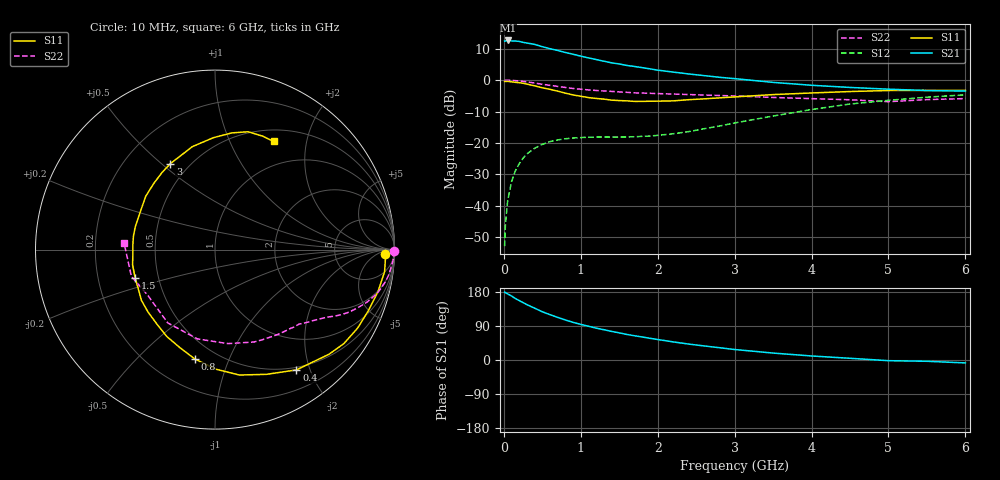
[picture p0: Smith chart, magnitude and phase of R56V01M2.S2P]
! SIEMENS Small Signal Semiconductors
! BFR183
! Si NPN RF Bipolar Junction Transistor in SOT23
! VCE = 6 V  IC = 1.2 mA
! Common Emitter S-Parameters:  May  1996
# GHz  S  MA  R  50
!  f  S11  S21  S12  S22
! GHz  MAG  ANG  MAG  ANG  MAG  ANG  MAG  ANG
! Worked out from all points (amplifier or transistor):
!   36 points, 10 MHz to 6 GHz, reference 50 ohm
!   highest |S21| = 12.6 dB at 50 MHz (marker M1)
!   |S21| within 3 dB of that: start of sweep to 669 MHz
!   unconditionally stable (mu >= 1): 1.618 GHz to 2.906 GHz
!   at 250 MHz: K = 0.16, MSG = 18.4 dB, |S12| = -24.8 dB
!   at 1.4 GHz: K = 0.89, MSG = 11.8 dB, |S12| = -18.1 dB
!   at 6 GHz: K = 0.93, MSG = 0.6 dB, |S12| = -4.7 dB
!   S11 on the Smith chart (normalised r, x): 10 MHz: 31, -15; 400 MHz: 0.46, -1.79; 800 MHz: 0.38, -0.76; 1.5 GHz: 0.37, -0.15; 3 GHz: 0.40, +0.53; 6 GHz: 0.65, +1.47
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0.01  0.9488 -1.4  4.147 179.2  0.0023 88.4  0.998 -0.5
0.02  0.9509 -2.9  4.182 177.6  0.005 88.0  0.9928 -1.0
0.05  0.9529 -7.4  4.253 174.4  0.0122 86.0  0.9962 -2.8
0.1  0.9376 -14.5  4.18 168.9  0.0243 82.0  0.9872 -5.4
0.15  0.9196 -21.8  4.165 162.2  0.0362 76.4  0.9787 -8.2
0.2  0.9071 -28.8  4.107 156.8  0.0469 72.7  0.9665 -10.6
0.3  0.8624 -42.5  3.875 146.1  0.0672 65.7  0.9359 -15.1
0.4  0.8094 -55.9  3.688 136.8  0.0825 58.6  0.896 -19.1
0.5  0.7522 -67.5  3.386 127.3  0.0952 53.0  0.8563 -22.4
0.6  0.7119 -79.0  3.146 119.7  0.1053 48.1  0.8241 -25.0
0.8  0.6195 -100.5  2.739 105.6  0.1168 40.9  0.7622 -29.1
0.9  0.5798 -109.8  2.57 99.4  0.1201 38.7  0.7349 -30.7
1.1  0.5262 -128.0  2.249 89.1  0.1236 35.6  0.6973 -33.7
1.2  0.5104 -136.9  2.116 84.1  0.1244 34.5  0.683 -35.1
1.5  0.472 -160.4  1.8 71.6  0.1244 35.2  0.6484 -38.9
1.7  0.458 -177.2  1.642 63.9  0.1255 38.2  0.6261 -41.5
2.2  0.4668 152.8  1.339 47.8  0.1401 47.8  0.599 -49.3
3  0.5394 117.5  1.053 27.7  0.208 56.7  0.5591 -67.0
3.5  0.5874 102.4  0.918 18.3  0.2681 55.0  0.5287 -82.2
4.5  0.6569 81.8  0.763 4.5  0.4161 43.1  0.4859 -122.8
5.5  0.6855 67.2  0.681 -3.4  0.5347 26.7  0.4891 -162.2
6  0.6853 61.6  0.668 -7.7  0.5827 16.8  0.5079 175.8
